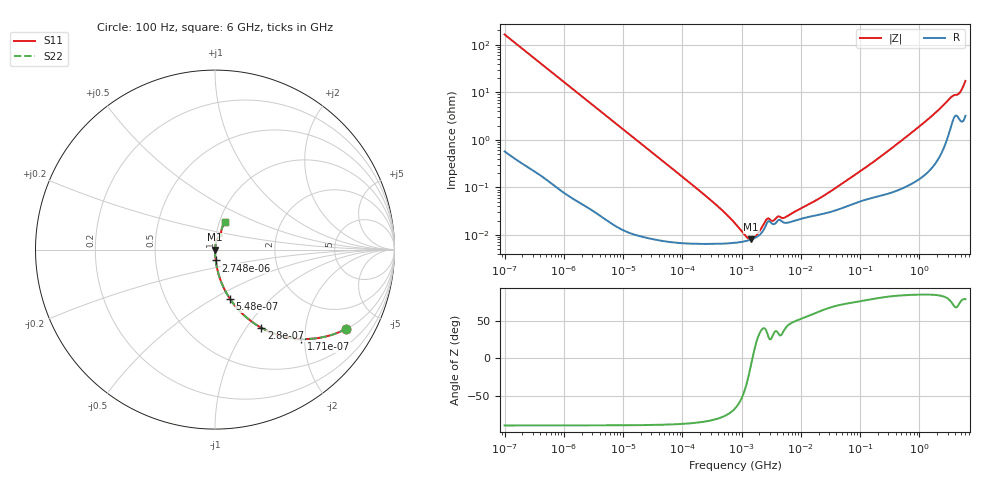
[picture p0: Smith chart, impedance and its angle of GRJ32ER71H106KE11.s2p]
!Murata Part Number: GRJ32ER71H106KE11
!These Parameters are Measured in Series Mode Connection
!Data Generated on Jun 19, 2026
!  o--ll--o
!Port1  Port2
!  o------o
!Operation Temp=25[degC], DC Bias Voltage=0[V]
!Freq. Start=100[Hz] Stop=6[GHz] 401[Steps]
# Hz S RI R 50
!Freq.(Hz) S11(Real) S11(Imag) S21(Real) S21(Imag) S12(Real) S12(Imag) S22(Real) S22(Imag)
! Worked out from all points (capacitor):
!   401 points, 100 Hz to 6 GHz, reference 50 ohm
!   read as one part in series: C = 9.65 uF near 109 Hz
!   lowest |Z| = 8.07 mohm at 1.45 MHz (marker M1)
!   series resonance near 1.522 MHz, so ESL is about 1.1 nH
!   S11 on the Smith chart (normalised r, x): 100 Hz: 1.01, -3.29; 171 Hz: 1.01, -1.93; 280 Hz: 1.00, -1.18; 548 Hz: 1.00, -0.60; 2.748 kHz: 1.00, -0.12; 6 GHz: 1.06, +0.34
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100  0.73 -0.4422  0.27 0.4422  0.27 0.4422  0.73 -0.4422
171  0.4816 -0.4978  0.5184 0.4978  0.5184 0.4978  0.4816 -0.4978
280  0.2588 -0.436  0.7412 0.436  0.7412 0.436  0.2588 -0.436
548  0.0845 -0.2759  0.9155 0.2759  0.9155 0.2759  0.0845 -0.2759
2008  0.00722 -0.082  0.9928 0.082  0.9928 0.082  0.00722 -0.082
2748  0.00399 -0.0602  0.996 0.0602  0.996 0.0602  0.00399 -0.0602
40335  9.39e-05 -0.00415  0.9999 0.00415  0.9999 0.00415  9.39e-05 -0.00415
316350  6.49e-05 -0.000508  0.9999 0.000508  0.9999 0.000508  6.49e-05 -0.000508
774597  6.81e-05 -0.000161  0.9999 0.000161  0.9999 0.000161  6.81e-05 -0.000161
1108252  7.29e-05 -7.19e-05  0.9999 7.19e-05  0.9999 7.19e-05  7.29e-05 -7.19e-05
1449809  7.99e-05 -1.1e-05  0.9999 1.1e-05  0.9999 1.1e-05  7.99e-05 -1.1e-05
1896632  9.45e-05 5.16e-05  0.9999 -5.16e-05  0.9999 -5.16e-05  9.45e-05 5.16e-05
2713602  0.000182 0.000122  0.9998 -0.000122  0.9998 -0.000122  0.000182 0.000122
3394479  0.000168 0.000103  0.9998 -0.000103  0.9998 -0.000103  0.000168 0.000103
5311619  0.00018 0.000144  0.9998 -0.000144  0.9998 -0.000144  0.00018 0.000144
1.555665e7  0.000248 0.000411  0.9998 -0.000411  0.9998 -0.000411  0.000248 0.000411
7.129496e7  0.000436 0.00157  0.9996 -0.00157  0.9996 -0.00157  0.000436 0.00157
3.124326e8  0.000786 0.00606  0.9992 -0.00606  0.9992 -0.00606  0.000786 0.00606
1.369159e9  0.00272 0.0262  0.9973 -0.0262  0.9973 -0.0262  0.00272 0.0262
3.352442e9  0.0222 0.0716  0.9778 -0.0716  0.9778 -0.0716  0.0222 0.0716
4.586474e9  0.0351 0.0818  0.9649 -0.0818  0.9649 -0.0818  0.0351 0.0818
6e9  0.0568 0.1561  0.9432 -0.1561  0.9432 -0.1561  0.0568 0.1561
